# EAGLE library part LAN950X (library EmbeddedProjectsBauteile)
Hi-Speed USB 2.0 to 10/100 Ethernet Controller
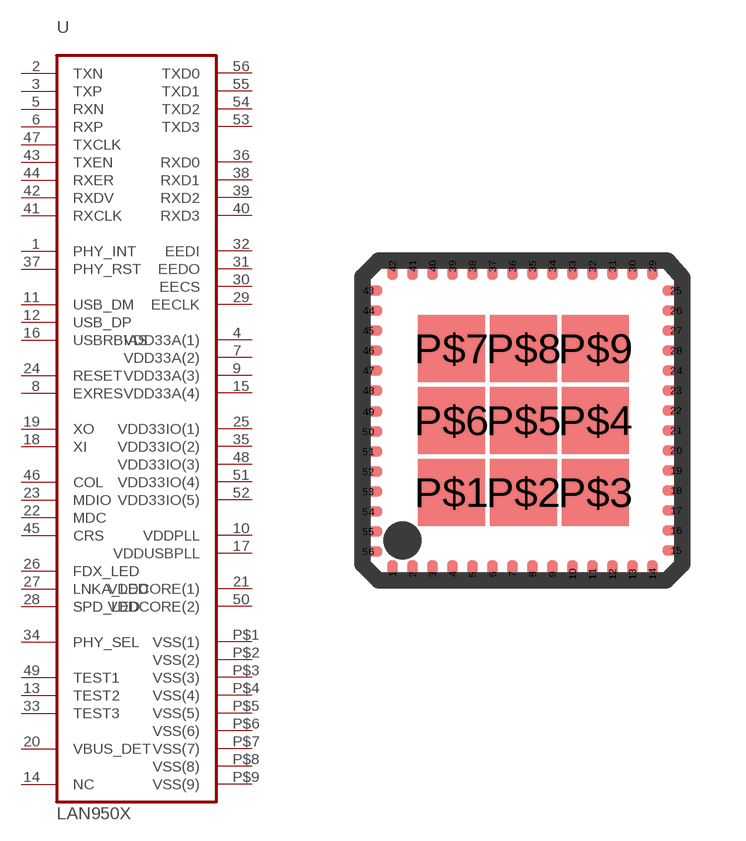
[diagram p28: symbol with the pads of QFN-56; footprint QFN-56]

Designator prefix -

## LAN950X (EP: 400468)  [QFN-56]
1  PHY_INT
2  TXN
3  TXP
4  VDD33A(1)  pwr
5  RXN
6  RXP
7  VDD33A(2)  pwr
8  EXRES  in
9  VDD33A(3)  pwr
10  VDDPLL  pwr
11  USB_DM
12  USB_DP
13  TEST2
14  NC  nc
15  VDD33A(4)  pwr
16  USBRBIAS  in
17  VDDUSBPLL
18  XI  in
19  XO  out
20  VBUS_DET  in
21  VDDCORE(1)  pwr
22  MDC
23  MDIO
24  RESET  in
25  VDD33IO(1)  pwr
26  FDX_LED
27  LNKA_LED
28  SPD_LED
29  EECLK
30  EECS  out
31  EEDO  out
32  EEDI  in
33  TEST3
34  PHY_SEL
35  VDD33IO(2)  pwr
36  RXD0  in
37  PHY_RST  in
38  RXD1  in
39  RXD2  in
40  RXD3  in
41  RXCLK  in
42  RXDV  in
43  TXEN
44  RXER  in
45  CRS
46  COL
47  TXCLK  out
48  VDD33IO(3)  pwr
49  TEST1
50  VDDCORE(2)  pwr
51  VDD33IO(4)
52  VDD33IO(5)
53  TXD3
54  TXD2
55  TXD1
56  TXD0
P$1  VSS(1)  pwr
P$2  VSS(2)  pwr
P$3  VSS(3)  pwr
P$4  VSS(4)  pwr
P$5  VSS(5)  pwr
P$6  VSS(6)  pwr
P$7  VSS(7)  pwr
P$8  VSS(8)
P$9  VSS(9)

## Footprint QFN-56 (pad centres in mm)
smd 0.27 x 0.7: 1 0.92,0.35; 2 1.42,0.35; 3 1.92,0.35; 4 2.42,0.35; 5 2.92,0.35; 6 3.42,0.35; 7 3.92,0.35; 8 4.42,0.35; 9 4.92,0.35; 10 5.42,0.35; 11 5.92,0.35; 12 6.42,0.35; 13 6.92,0.35; 14 7.42,0.35; 29 7.42,8.06; 30 6.92,8.06; 31 6.42,8.06; 32 5.92,8.06; 33 5.42,8.06; 34 4.92,8.06; 35 4.42,8.06; 36 3.92,8.06; 37 3.42,8.06; 38 2.92,8.06; 39 2.42,8.06; 40 1.92,8.06; 41 1.42,8.06; 42 0.92,8.06
smd 0.7 x 0.27: 15 8.02,0.95; 16 8.02,1.45; 17 8.02,1.95; 18 8.02,2.45; 19 8.02,2.95; 20 8.02,3.45; 21 8.02,3.95; 22 8.02,4.45; 23 8.02,4.95; 24 8.02,5.45; 25 8.02,7.45; 26 8.02,6.95; 27 8.02,6.45; 28 8.02,5.95; 43 0.32,7.45; 44 0.32,6.95; 45 0.32,6.45; 46 0.32,5.95; 47 0.32,5.45; 48 0.32,4.95; 49 0.32,4.42; 50 0.32,3.92; 51 0.32,3.42; 52 0.32,2.92; 53 0.32,2.42; 54 0.32,1.92; 55 0.32,1.42; 56 0.32,0.92
smd 1.676 x 1.676: P$1 2.4,2.4; P$2 4.2,2.4; P$3 6,2.4; P$4 6,4.2; P$5 4.2,4.2; P$6 2.4,4.2; P$7 2.4,6; P$8 4.2,6; P$9 6,6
